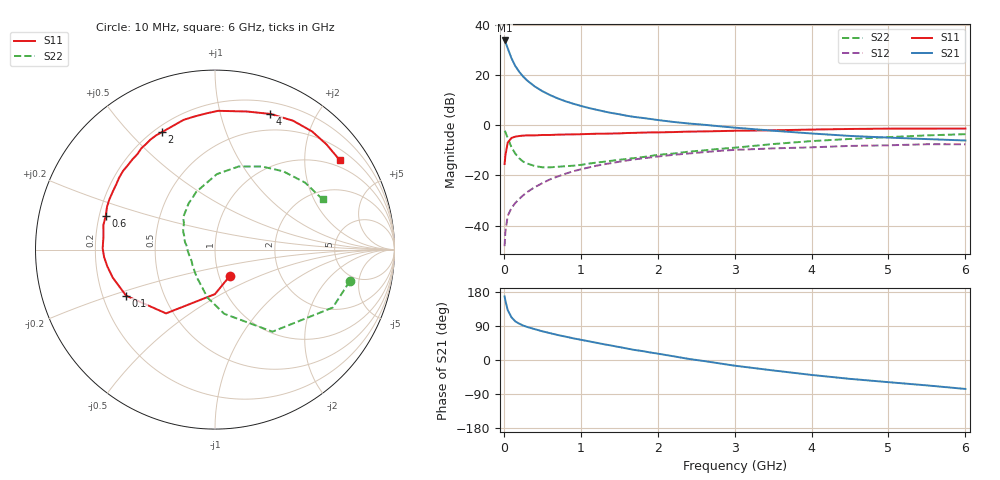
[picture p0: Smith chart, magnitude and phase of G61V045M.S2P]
! SIEMENS Small Signal Semiconductors
! BFG193
! Si NPN RF Bipolar Junction Transistor in SOT223
! VCE = 1 V  IC = 45 mA
! Common Emitter S-Parameters:  August  1996
# GHz  S  MA  R  50
!  f  S11  S21  S12  S22
! GHz  MAG  ANG  MAG  ANG  MAG  ANG  MAG  ANG
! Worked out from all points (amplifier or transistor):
!   36 points, 10 MHz to 6 GHz, reference 50 ohm
!   highest |S21| = 33.7 dB at 10 MHz (marker M1)
!   |S21| within 3 dB of that: start of sweep to 48.96 MHz
!   unconditionally stable (mu >= 1): start of sweep to 10.54 MHz; 270.9 MHz to 4.464 GHz; 5.515 GHz to end of sweep
!   at 250 MHz: K = 0.99, MSG = 23.7 dB, |S12| = -28.0 dB
!   at 1.4 GHz: K = 1.12, MAG = 7.9 dB, |S12| = -15.1 dB
!   at 6 GHz: K = 1.01, MAG = 0.2 dB, |S12| = -7.6 dB
!   S11 on the Smith chart (normalised r, x): 10 MHz: 1.13, -0.34; 100 MHz: 0.30, -0.22; 600 MHz: 0.23, +0.14; 2 GHz: 0.23, +0.62; 4 GHz: 0.32, +1.44; 6 GHz: 0.79, +2.92
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0.01  0.1683 -60.4  48.51 167.6  0.0039 78.2  0.7714 -13.2
0.02  0.2482 -90.1  45.31 156.7  0.0075 75.0  0.7312 -26.2
0.05  0.448 -127.5  34 131.8  0.0156 60.2  0.5583 -55.0
0.1  0.558 -152.6  21.34 112.5  0.0225 57.8  0.3613 -81.8
0.15  0.5908 -164.7  14.95 101.8  0.0284 58.0  0.2699 -99.1
0.2  0.6076 -171.3  11.54 95.8  0.0341 60.3  0.2186 -109.8
0.25  0.6192 -176.1  9.299 91.1  0.0399 61.6  0.1887 -121.1
0.3  0.6259 179.4  7.809 87.4  0.0461 62.7  0.1732 -128.9
0.4  0.6258 173.2  5.917 81.5  0.0581 63.9  0.1539 -143.9
0.5  0.6369 167.5  4.752 75.8  0.07 63.2  0.1449 -154.9
0.6  0.637 162.8  3.974 70.9  0.0833 62.5  0.1446 -163.0
0.8  0.6516 154.7  2.992 61.7  0.1076 59.0  0.1523 -178.0
1.1  0.6676 143.2  2.204 49.5  0.1433 53.4  0.171 166.6
1.6  0.6978 126.0  1.537 30.3  0.198 41.4  0.213 146.1
2  0.7182 114.2  1.266 16.8  0.2373 31.6  0.256 133.1
2.2  0.7277 108.9  1.161 10.0  0.2561 26.7  0.2716 126.7
2.8  0.7609 93.4  0.951 -8.8  0.3076 11.9  0.337 108.3
3.5  0.7896 77.0  0.775 -27.5  0.3448 -6.2  0.4206 88.6
4  0.8164 67.8  0.683 -39.4  0.362 -15.8  0.4816 74.1
4.5  0.8395 58.8  0.61 -49.8  0.3859 -25.7  0.5314 60.6
5.5  0.8541 43.4  0.528 -67.0  0.4171 -48.1  0.6257 36.6
6  0.8554 35.6  0.495 -76.4  0.416 -60.8  0.6615 25.0
